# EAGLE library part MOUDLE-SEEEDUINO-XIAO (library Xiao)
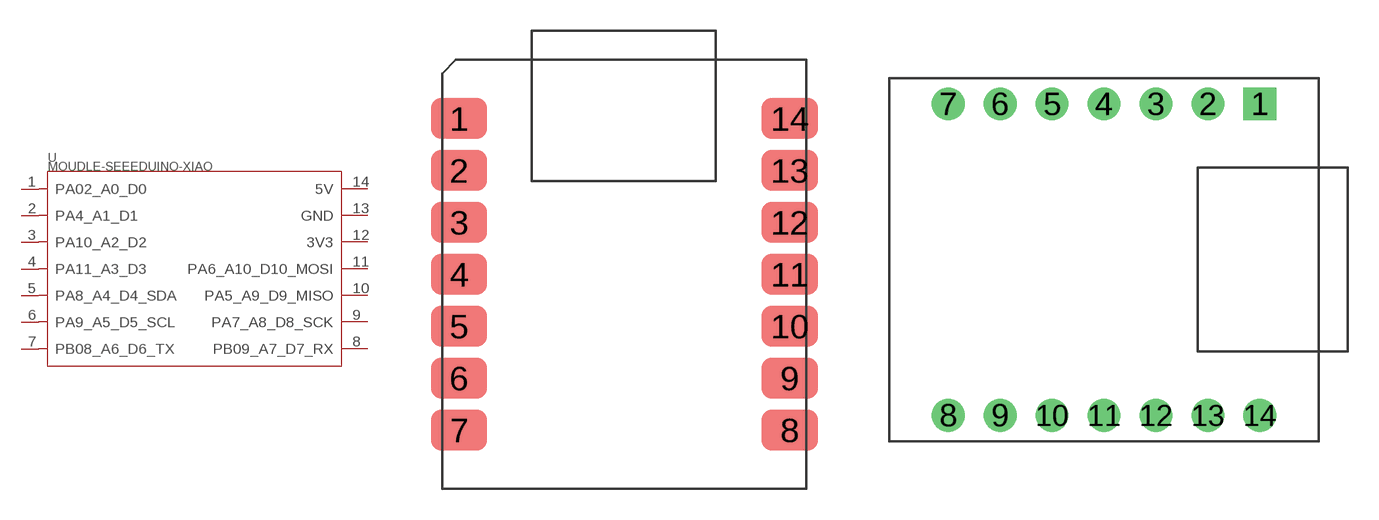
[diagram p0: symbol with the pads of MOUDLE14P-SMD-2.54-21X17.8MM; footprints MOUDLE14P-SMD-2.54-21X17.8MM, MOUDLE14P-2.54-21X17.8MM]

Designator prefix U

## MOUDLE-SEEEDUINO-XIAO-SMD  [MOUDLE14P-SMD-2.54-21X17.8MM]
1  PA02_A0_D0
2  PA4_A1_D1
3  PA10_A2_D2
4  PA11_A3_D3
5  PA8_A4_D4_SDA
6  PA9_A5_D5_SCL
7  PB08_A6_D6_TX
8  PB09_A7_D7_RX
9  PA7_A8_D8_SCK
10  PA5_A9_D9_MISO
11  PA6_A10_D10_MOSI
12  3V3
13  GND
14  5V

## MOUDLE-SEEEDUINO-XIAO-DIP  [MOUDLE14P-2.54-21X17.8MM]
Pads as for MOUDLE14P-SMD-2.54-21X17.8MM

## Footprint MOUDLE14P-SMD-2.54-21X17.8MM (pad centres in mm)
smd 2.75 x 2: 1 0.835,18.12; 2 0.835,15.58; 3 0.835,13.04; 4 0.835,10.5; 5 0.835,7.96; 6 0.835,5.42; 7 0.835,2.88; 8 17,2.88; 9 17,5.42; 10 17,7.96; 11 17,10.5; 12 17,13.04; 13 17,15.58; 14 17,18.12

## Footprint MOUDLE14P-2.54-21X17.8MM (pad centres in mm)
drill 1 pad 1.6 square: 1 7.62,7.62
drill 1 pad 1.6: 2 5.08,7.62; 3 2.54,7.62; 4 0,7.62; 5 -2.54,7.62; 6 -5.08,7.62; 7 -7.62,7.62; 8 -7.62,-7.62; 9 -5.08,-7.62; 10 -2.54,-7.62; 11 0,-7.62; 12 2.54,-7.62; 13 5.08,-7.62; 14 7.62,-7.62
